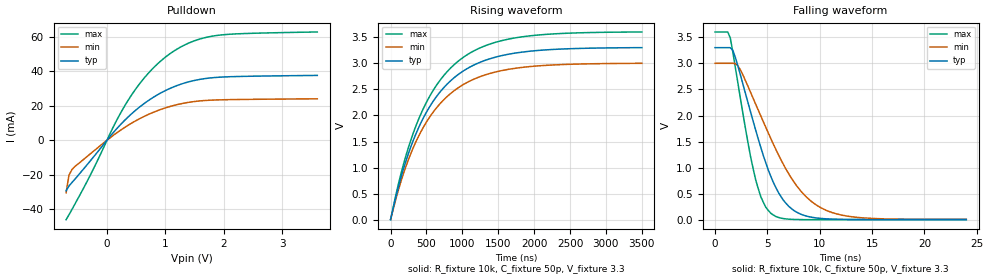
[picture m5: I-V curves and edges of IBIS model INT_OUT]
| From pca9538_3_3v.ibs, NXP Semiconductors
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[Model]   INT_OUT
Model_type Open_drain
Vref=3.3
Vmeas=1.65
Rref=10k
Cref=50p
C_comp   5.2p   5p   5.4p
[Temperature Range] 27   85   -40
[Voltage Range]   3.3   3   3.6
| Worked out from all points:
|   slope of the pulldown table from 0 to 0.495 V, typ, clamps not added: 28.2 ohm
|   falling waveform, R_fixture 10k, C_fixture 50p, V_fixture 3.3: 20-80 % time 3.09ns typ, 4.49ns min, 1.98ns max; typ from 3.3 V to 0.008 V
|   rising waveform, R_fixture 10k, C_fixture 50p, V_fixture 3.3: 20-80 % time 702ns typ, 703ns min, 701ns max; typ from 0.008 V to 3.3 V
[Pulldown]
-700mV    -29.34mA   -30.57mA   -46.16mA
-650mV    -26.57mA   -20.28mA   -43.28mA
-600mV    -24.56mA   -17.03mA   -40.24mA
-250mV    -10.52mA   -6.91mA    -17.88mA
150mV     6.068mA    3.88mA     10.55mA
350mV     13.13mA    8.458mA    22.56mA
500mV     17.69mA    11.45mA    30.15mA
700mV     22.87mA    14.86mA    38.63mA
1.05V     29.66mA    19.33mA    49.58mA
1.45V     34.38mA    22.29mA    57.17mA
1.85V     36.45mA    23.38mA    60.73mA
3.6V      37.67mA    24.07mA    62.9mA
[Falling Waveform]
R_fixture=10k
C_fixture=50p
V_fixture=3.3
V_fixture_min=3
V_fixture_max=3.6
0s        3.3V       3V         3.6V
1.455ns   3.299V     3V         3.485V
2.182ns   2.949V     2.952V     2.62V
3.879ns   1.722V     2.218V     769.2mV
4.364ns   1.393V     1.994V     447.5mV
5.333ns   832.4mV    1.556V     126.7mV
6.545ns   372.9mV    1.058V     25.84mV
7.515ns   182.6mV    734.5mV    9.656mV
10.67ns   21.08mV    179.8mV    4.868mV
24ns      7.773mV    11.27mV    4.826mV
[Rising Waveform]
R_fixture=10k
C_fixture=50p
V_fixture=3.3
V_fixture_min=3
V_fixture_max=3.6
0s        7.771mV    11.11mV    4.827mV
106.1ns   613.2mV    558.2mV    668.8mV
212.1ns   1.118V     1.016V     1.221V
318.2ns   1.529V     1.389V     1.67V
424.2ns   1.863V     1.692V     2.034V
671.7ns   2.417V     2.196V     2.639V
989.9ns   2.829V     2.57V      3.088V
1.343us   3.065V     2.786V     3.345V
1.803us   3.205V     2.913V     3.497V
3.5us     3.296V     2.996V     3.596V
[Ramp]
R_load=10k
dV/dt_r   1.776E+0/8.850E-9   1.716E+0/9.131E-9   1.837E+0/8.389E-9
dV/dt_f   1.975E+0/1.440E-10   1.973E+0/2.182E-10   1.977E+0/7.953E-11
|[End   INT_OUT
